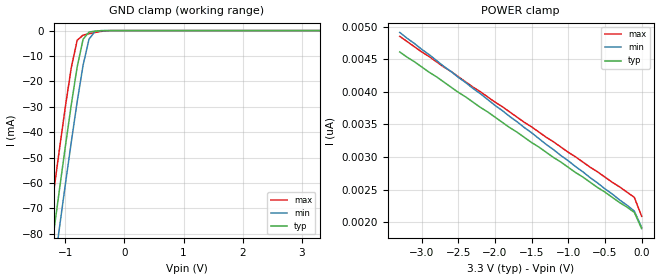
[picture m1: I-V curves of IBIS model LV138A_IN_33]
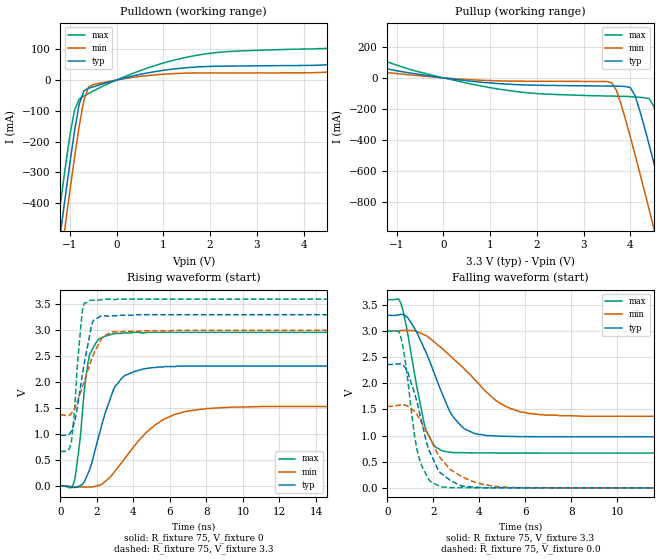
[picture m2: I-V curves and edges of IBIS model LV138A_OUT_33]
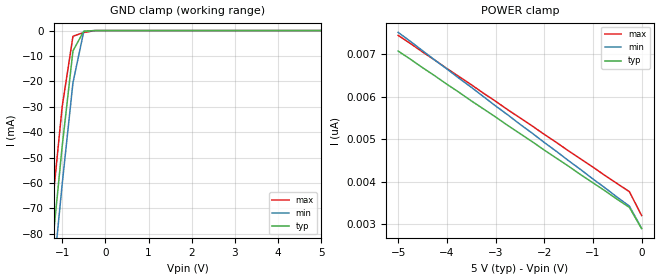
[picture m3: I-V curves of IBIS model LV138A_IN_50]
| TEXAS INSTRUMENTS INCORPORATED
| Standard Linear and Logic Group
| IBIS Model of SN74LV138A
| 3-LINE TO 8-LINE DECODER/DEMULTIPLEXER
| SOIC 16-pin (D), SOP 16-pin (NS), SSOP 16-pin (DB), TSSOP 16-pin (PW)
| and TVSOP 16-pin (DGV) Package
[IBIS Ver]   3.2
[Comment Char]  |_char
[File Name]   lv138a.ibs
[File Rev]   2.0 H_die
[Date]   May 26, 2000
[Source]   Data created from HSPICE simulations at TI-SLL.
[Notes]   The following is an IBIS list for the LV138A.
|   Please contact sllibis@ti.com with questions and
|   comments concerning SLL IBIS models.
|   The warning about AC Rising Endpoint might be reported,
|   but it is due to HSPICE issue and negligible.
[Disclaimer] Property of Texas Instruments Incorporated.  Unauthorized
   reproduction and/or distribution is strictly prohibited.
   This product is protected under copyright law.
   Created 2000, (C) Copyright 2000, Texas Instruments Inc.,
   All Rights Reserved.
   UNLESS THERE IS A SIGNED, WRITTEN AGREEMENT TO THE
   CONTRARY, TEXAS INSTRUMENTS () IS PROVIDING THE IBIS
   MODELS  AND WITHOUT ANY WARRANTY, EXPRESSED OR
   IMPLIED.  TI assumes no liability for:
   1) the accuracy of the IBIS models provided to your
   company;
   2) the proper functioning of these IBIS Models in your
   design or for any resulting applications; or
   3) infringement of patents, copyrights or intellectual
   property rights resulting from your use of these IBIS
   models.
   TI provides IBIS Models as a service to our customers.
   You and your company shall not distribute, sell or give
   these models to anyone else without prior written
   permission from TI.
   TI reserves the right to make changes to our products or
   to discontinue any semiconductor product or service
   without notice, and advises our customers to obtain the
   latest version of relevant information to verify, before
   placing orders, that the information being relied on is
   current.
   Please be aware that your receipt and use of the IBIS
   information provided shall serve as acceptance of these
   terms and conditions.  If you do not accept these terms,
   you should return or destroy the IBIS models and any
   other accompanying information immediately.
|   Component LV138A_D
[Component]   LV138A_D
[Manufacturer]  Texas Instruments, Inc.
[Package]
|   typ   min   max
R_pkg   0.039   0.028   0.049
L_pkg   3.453nH   2.350nH   4.375nH
C_pkg   0.521pF   0.254pF   0.708pF
[Pin]   signal_name   model_name   R_pin   L_pin   C_pin
1   A   LV138A_IN   0.042   4.336nH   0.703pF
2   B   LV138A_IN   0.049   3.778nH   0.634pF
3   C   LV138A_IN   0.028   3.449nH   0.518pF
4   G2A_NOT   LV138A_IN   0.029   2.393nH   0.254pF
5   G2B_NOT   LV138A_IN   0.028   2.350nH   0.264pF
6   G1   LV138A_IN   0.048   3.312nH   0.483pF
7   Y7   LV138A_OUT   0.043   3.629nH   0.604pF
8   GND   GND   0.044   4.375nH   0.708pF
9   Y6   LV138A_OUT   0.042   4.336nH   0.703pF
10   Y5   LV138A_OUT   0.049   3.778nH   0.634pF
11   Y4   LV138A_OUT   0.028   3.449nH   0.518pF
12   Y3   LV138A_OUT   0.029   2.393nH   0.255pF
13   Y2   LV138A_OUT   0.028   2.350nH   0.264pF
14   Y1   LV138A_OUT   0.048   3.312nH   0.483pF
15   Y0   LV138A_OUT   0.043   3.629nH   0.604pF
16   VCC   POWER   0.044   4.375nH   0.708pF
|   Component LV138A_NS
[Component]   LV138A_NS
[Manufacturer]  Texas Instruments, Inc.
[Package]
|   typ   min   max
R_pkg   0.042   0.035   0.049
L_pkg   3.147nH   2.164nH   4.219nH
C_pkg   0.404pF   0.241pF   0.562pF
[Pin]   signal_name   model_name   R_pin   L_pin   C_pin
1   A   LV138A_IN   0.049   4.215nH   0.562pF
2   B   LV138A_IN   0.046   3.675nH   0.480pF
3   C   LV138A_IN   0.037   2.527nH   0.332pF
4   G2A_NOT   LV138A_IN   0.035   2.164nH   0.241pF
5   G2B_NOT   LV138A_IN   0.035   2.164nH   0.241pF
6   G1   LV138A_IN   0.037   2.527nH   0.332pF
7   Y7   LV138A_OUT   0.046   3.675nH   0.480pF
8   GND   GND   0.049   4.215nH   0.562pF
9   Y6   LV138A_OUT   0.049   4.219nH   0.562pF
10   Y5   LV138A_OUT   0.046   3.679nH   0.480pF
11   Y4   LV138A_OUT   0.037   2.531nH   0.333pF
12   Y3   LV138A_OUT   0.035   2.168nH   0.241pF
13   Y2   LV138A_OUT   0.035   2.168nH   0.241pF
14   Y1   LV138A_OUT   0.037   2.531nH   0.333pF
15   Y0   LV138A_OUT   0.046   3.679nH   0.480pF
16   VCC   POWER   0.049   4.219nH   0.562pF
|   Component LV138A_DB
[Component]   LV138A_DB
[Manufacturer]  Texas Instruments, Inc.
[Package]
|   typ   min   max
R_pkg   0.048   0.046   0.050
L_pkg   3.536nH   3.213nH   3.798nH
C_pkg   0.376pF   0.314pF   0.440pF
[Pin]   signal_name   model_name   R_pin   L_pin   C_pin
1   A   LV138A_IN   0.048   3.797nH   0.377pF
2   B   LV138A_IN   0.046   3.723nH   0.440pF
3   C   LV138A_IN   0.048   3.409nH   0.372pF
4   G2A_NOT   LV138A_IN   0.049   3.213nH   0.314pF
5   G2B_NOT   LV138A_IN   0.049   3.213nH   0.314pF
6   G1   LV138A_IN   0.048   3.409nH   0.372pF
7   Y7   LV138A_OUT   0.046   3.723nH   0.440pF
8   GND   GND   0.048   3.798nH   0.377pF
9   Y6   LV138A_OUT   0.048   3.797nH   0.377pF
10   Y5   LV138A_OUT   0.046   3.725nH   0.440pF
11   Y4   LV138A_OUT   0.048   3.409nH   0.372pF
12   Y3   LV138A_OUT   0.049   3.214nH   0.314pF
13   Y2   LV138A_OUT   0.050   3.216nH   0.314pF
14   Y1   LV138A_OUT   0.048   3.409nH   0.372pF
15   Y0   LV138A_OUT   0.047   3.729nH   0.440pF
16   VCC   POWER   0.048   3.797nH   0.377pF
|   Component LV138A_PW
[Component]   LV138A_PW
[Manufacturer]  Texas Instruments, Inc.
[Package]
|   typ   min   max
R_pkg   0.045   0.038   0.051
L_pkg   2.593nH   2.447nH   3.080nH
C_pkg   0.281pF   0.243pF   0.377pF
[Pin]   signal_name   model_name   R_pin   L_pin   C_pin
1   A   LV138A_IN   0.040   3.080nH   0.377pF
2   B   LV138A_IN   0.038   2.458nH   0.281pF
3   C   LV138A_IN   0.051   2.512nH   0.255pF
4   G2A_NOT   LV138A_IN   0.051   2.447nH   0.243pF
5   G2B_NOT   LV138A_IN   0.051   2.447nH   0.243pF
6   G1   LV138A_IN   0.051   2.512nH   0.255pF
7   Y7   LV138A_OUT   0.038   2.458nH   0.281pF
8   GND   GND   0.040   3.080nH   0.377pF
9   Y6   LV138A_OUT   0.039   2.832nH   0.316pF
10   Y5   LV138A_OUT   0.038   2.460nH   0.279pF
11   Y4   LV138A_OUT   0.051   2.512nH   0.255pF
12   Y3   LV138A_OUT   0.051   2.447nH   0.243pF
13   Y2   LV138A_OUT   0.051   2.447nH   0.243pF
14   Y1   LV138A_OUT   0.051   2.512nH   0.255pF
15   Y0   LV138A_OUT   0.038   2.459nH   0.279pF
16   VCC   POWER   0.039   2.832nH   0.316pF
|   Component LV138A_DGV
[Component]   LV138A_DGV
[Manufacturer]  Texas Instruments, Inc.
[Package]
|   typ   min   max
R_pkg   0.039   0.033   0.045
L_pkg   2.543nH   2.320nH   2.938nH
C_pkg   0.386pF   0.334pF   0.449pF
[Pin]   signal_name   model_name   R_pin   L_pin   C_pin
1   A   LV138A_IN   0.035   2.907nH   0.417pF
2   B   LV138A_IN   0.042   2.558nH   0.446pF
3   C   LV138A_IN   0.038   2.341nH   0.345pF
4   G2A_NOT   LV138A_IN   0.038   2.320nH   0.334pF
5   G2B_NOT   LV138A_IN   0.039   2.322nH   0.334pF
6   G1   LV138A_IN   0.038   2.353nH   0.342pF
7   Y7   LV138A_OUT   0.040   2.536nH   0.441pF
8   GND   GND   0.033   2.897nH   0.418pF
9   Y6   LV138A_OUT   0.035   2.927nH   0.419pF
10   Y5   LV138A_OUT   0.045   2.632nH   0.449pF
11   Y4   LV138A_OUT   0.039   2.368nH   0.347pF
12   Y3   LV138A_OUT   0.039   2.330nH   0.335pF
13   Y2   LV138A_OUT   0.039   2.320nH   0.335pF
14   Y1   LV138A_OUT   0.039   2.361nH   0.345pF
15   Y0   LV138A_OUT   0.041   2.573nH   0.446pF
16   VCC   POWER   0.035   2.938nH   0.420pF
[Model Selector]   LV138A_IN
LV138A_IN_33   3.3-V Vcc Input Model
LV138A_IN_50   5.0-V Vcc Input Model
[Model Selector]   LV138A_OUT
LV138A_OUT_33   3.3-V Vcc Output Model
LV138A_OUT_50   5.0-V Vcc Output Model
| Models and submodels in the file (4): LV138A_IN_33 (Input), LV138A_OUT_33 (Output), LV138A_IN_50 (Input), LV138A_OUT_50 (Output)
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|   Model LV138A_IN_33
[Model]   LV138A_IN_33
Model_type  Input
Polarity   Inverting
Vinl = 0.99
Vinh = 2.31
| variable   typ   min   max
C_comp   1.35pf   1.01pf   1.69pf
[Temperature Range]   25   85   -40
[Voltage Range]   3.3   3.0   3.6
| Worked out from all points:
|   GND clamp passes 1 mA (typ) near -0.61 V on its own axis
[GND Clamp]
|   Voltage   I(typ)   I(min)   I(max)
-3.3V     -460mA     -475mA     -445mA
-1.3V     -97.5mA    -113mA     -81.5mA
-1.2V     -79.9mA    -95mA      -63.9mA
-1.1V     -62.6mA    -77.6mA    -46.7mA
-1V       -45.6mA    -60.5mA    -30mA
-900mV    -29.2mA    -43.9mA    -14.6mA
-800mV    -14.3mA    -28mA      -3.81mA
-700mV    -3.42mA    -13.6mA    -1.78mA
-600mV    -581uA     -3.4mA     -1.25mA
-500mV    -233uA     -353uA     -759uA
-400mV    -58.1uA    -21.9uA    -324uA
3.3V      1.9nA      2.34nA     1.69nA
[POWER Clamp]
|   Voltage   I(typ)   I(min)   I(max)
-3.3V     4.61nA     4.91nA     4.85nA
-3V       4.38nA     4.65nA     4.61nA
-100mV    2.15nA     2.17nA     2.38nA
0V        1.9nA      1.92nA     2.09nA
|   Model LV138A_OUT_33
[Model]   LV138A_OUT_33
Model_type  Output
Polarity   Non-Inverting
Vmeas = 1.65v
Cref = 15pf
| variable   typ   min   max
C_comp   4.62pf   3.47pf   5.77pf
[Temperature Range]   25   85   -40
[Voltage Range]   3.3   3.0   3.6
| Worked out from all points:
|   slope of the pulldown table from 0 to 0.495 V, typ, clamps not added: 27.3 ohm
|   slope of the pullup table from 0 to 0.495 V, typ, clamps not added: 27.2 ohm
|   rising waveform, R_fixture 75, V_fixture 0: 20-80 % time 1.17ns typ, 2.38ns min, 543ps max; typ from 0 V to 2.31 V
|   falling waveform, R_fixture 75, V_fixture 3.3: 20-80 % time 1.32ns typ, 2.29ns min, 735ps max; typ from 3.3 V to 0.976 V
|   rising waveform, R_fixture 75, V_fixture 3.3: 20-80 % time 669ps typ, 1.01ns min, 379ps max; typ from 0.976 V to 3.3 V
|   falling waveform, R_fixture 75, V_fixture 0.0: 20-80 % time 947ps typ, 1.39ns min, 578ps max; typ from 2.36 V to 0 V
[Pulldown]
|   Voltage   I(typ)   I(min)   I(max)
-3.3V     -3.04A     -3.13A     -2.95A
-1.3V     -615mA     -707mA     -518mA
-1.2V     -498mA     -591mA     -401mA
-1.1V     -383mA     -475mA     -288mA
-900mV    -167mA     -253mA     -98.6mA
-800mV    -79.1mA    -151mA     -61.7mA
-700mV    -35.5mA    -66.4mA    -51.9mA
-600mV    -26.8mA    -23.2mA    -43.9mA
-500mV    -22mA      -14.7mA    -35.8mA
1.6V      41.2mA     22.8mA     77.1mA
4.7V      52.1mA     27.5mA     106mA
6.6V      86.8mA     47.3mA     166mA
[Pullup]
|   Voltage   I(typ)   I(min)   I(max)
-3.3V     168mA      92.9mA     314mA
600mV     -21.6mA    -12.3mA    -39.7mA
3.6V      -52.9mA    -31.5mA    -117mA
3.8V      -54.2mA    -168mA     -119mA
4V        -62.6mA    -381mA     -121mA
4.1V      -115mA     -494mA     -123mA
4.4V      -429mA     -845mA     -133mA
4.5V      -544mA     -964mA     -182mA
4.8V      -899mA     -1.32A     -505mA
4.9V      -1.02A     -1.44A     -622mA
5.2V      -1.38A     -1.81A     -981mA
6.6V      -3.09A     -3.52A     -2.69A
[Ramp]
| variable   typ   min   max
dV/dt_r   1.40E+00/1.19E-09   9.38E-01/2.46E-09   1.78E+00/4.88E-10
dV/dt_f   1.41E+00/1.35E-09   9.88E-01/2.32E-09   1.77E+00/7.51E-10
R_load = 75
[Rising Waveform]
R_fixture = 75
V_fixture = 0
|   Time   V(typ)   V(min)   V(max)
0s        0V         0V         0V
700ps     -29.8mV    -16.7mV    25.3mV
1ns       -7.39mV    -19.8mV    680mV
1.3ns     73.7mV     -21.5mV    1.81V
1.6ns     312mV      -21mV      2.54V
2.4ns     1.34V      69.7mV     2.88V
3.5ns     2.12V      519mV      2.95V
5.2ns     2.28V      1.18V      2.96V
6.9ns     2.31V      1.44V      2.96V
25ns      2.31V      1.53V      2.96V
[Falling Waveform]
R_fixture = 75
V_fixture = 3.3
V_fixture_min = 3.0
V_fixture_max = 3.6
|   Time   V(typ)   V(min)   V(max)
0s        3.3V       3V         3.6V
600ps     3.32V      3.01V      3.52V
900ps     3.25V      3.01V      2.92V
1.6ns     2.67V      2.93V      1.24V
2ns       2.24V      2.81V      834mV
2.4ns     1.79V      2.66V      708mV
3.4ns     1.12V      2.25V      672mV
4.9ns     989mV      1.62V      667mV
6.2ns     979mV      1.42V      667mV
25ns      976mV      1.37V      666mV
[Rising Waveform]
R_fixture = 75
V_fixture = 3.3
V_fixture_min = 3.0
V_fixture_max = 3.6
|   Time   V(typ)   V(min)   V(max)
0s        976mV      1.37V      666mV
600ps     1.06V      1.4V       847mV
800ps     1.27V      1.51V      1.59V
900ps     1.45V      1.6V       2.2V
1.2ns     2.15V      1.9V       3.38V
1.6ns     2.9V       2.33V      3.57V
1.8ns     3.19V      2.53V      3.58V
2.3ns     3.28V      2.86V      3.59V
2.8ns     3.27V      2.97V      3.59V
25ns      3.3V       3V         3.6V
[Falling Waveform]
R_fixture = 75
V_fixture = 0.0
|   Time   V(typ)   V(min)   V(max)
0s        2.36V      1.56V      3V
600ps     2.37V      1.59V      2.87V
800ps     2.29V      1.58V      2.37V
1.2ns     1.79V      1.46V      958mV
1.5ns     1.25V      1.24V      418mV
1.8ns     737mV      998mV      165mV
2.4ns     257mV      525mV      15.5mV
3.7ns     16.5mV     126mV      1.4mV
5.2ns     750uV      11.6mV     762uV
25ns      12.7uV     568nV      12.2uV
|   Model LV138A_IN_50
[Model]   LV138A_IN_50
Model_type  Input
Polarity   Inverting
Vinl = 1.5
Vinh = 3.5
| variable   typ   min   max
C_comp   1.35pf   1.01pf   1.69pf
[Temperature Range]   25   85   -40
[Voltage Range]   5.0   4.5   5.5
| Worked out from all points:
|   GND clamp passes 1 mA (typ) near -0.52 V on its own axis
[GND Clamp]
|   Voltage   I(typ)   I(min)   I(max)
-5V       -773mA     -786mA     -758mA
-1.5V     -133mA     -148mA     -117mA
-1.25V    -88.7mA    -104mA     -72.7mA
-1V       -45.6mA    -60.5mA    -30mA
-750mV    -7.99mA    -20.5mA    -2.23mA
-500mV    -233uA     -353uA     -759uA
-250mV    -2.63nA    -182nA     -26.9uA
5V        2.9nA      3.64nA     2.54nA
[POWER Clamp]
|   Voltage   I(typ)   I(min)   I(max)
-5V       7.08nA     7.52nA     7.45nA
-1.5V     4.37nA     4.5nA      4.73nA
-250mV    3.4nA      3.43nA     3.77nA
0V        2.9nA      2.91nA     3.21nA
